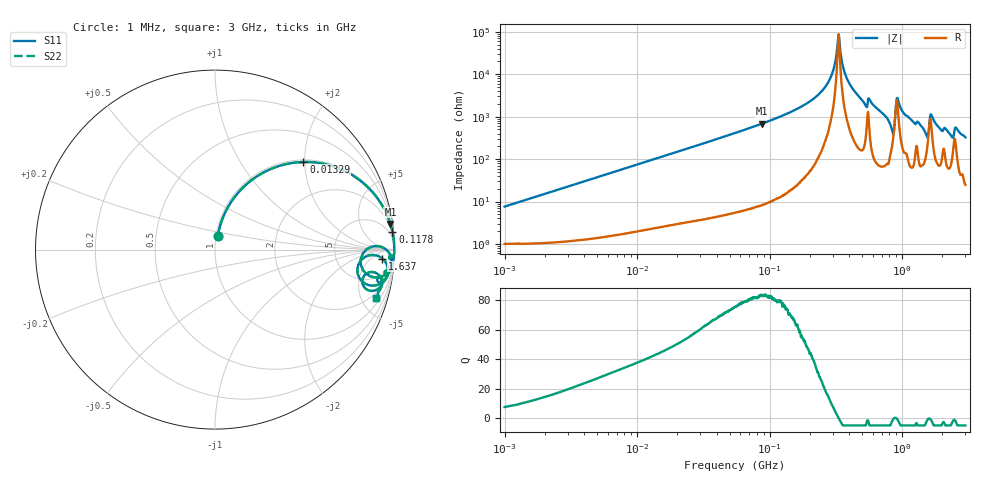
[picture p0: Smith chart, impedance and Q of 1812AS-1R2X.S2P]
!s-Parameter Generated by FASTRON Sdn. Bhd.
!FASTRON P/N : 1812AS-1R2X
!Keysight Technologies,E4991B,MY54100416,A.01.15
!Date created: Fri Oct 13 15:28:02 2023
!Version  : Rev00 Fri Oct 13 15:28:02 2023
!Data & Calibration Information:
!Freq	S11	S21	S12	S22
!PortZ  Port1:50+j0  Port2:50+j0
!When reading, reference impedance value at option line is always used.
! Remarks : This data is being provided solely for informational purposes.
# Hz S dB R 50
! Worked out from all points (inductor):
!   1601 points, 1 MHz to 3 GHz, reference 50 ohm
!   read as one part in series: L = 1.2 uH near 1.041 MHz
!   highest Q = 83.2 at 87.23 MHz (marker M1), where L = 1.25 uH
!   self-resonance near 330.2 MHz
!   S11 on the Smith chart (normalised r, x): 1 MHz: 1.02, +0.15; 13.29 MHz: 1.05, +1.97; 117.8 MHz: 1, +20; 1.637 GHz: 18, -14; 3 GHz: 1.50, -6.53
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1000000  -22.48 78.1  -0.11 -4.3  -0.11 -4.3  -22.48 78.1
3804036  -11.33 71.8  -0.44 -15.7  -0.44 -15.7  -11.33 71.8
1.329061e7  -3.18 44.7  -3.05 -43.9  -3.05 -43.9  -3.18 44.7
1.447069e7  -2.82 42.4  -3.42 -46.3  -3.42 -46.3  -2.82 42.4
5.477226e7  -0.28 13.6  -12.57 -75.6  -12.57 -75.6  -0.28 13.6
8.723049e7  -0.11 8.3  -16.79 -81.0  -16.79 -81.0  -0.11 8.3
1.17777e8  -0.06 5.8  -19.88 -83.5  -19.88 -83.5  -0.06 5.8
2.083556e8  -0.02 2.3  -27.90 -86.3  -27.90 -86.3  -0.02 2.3
2.827291e8  -0.01 0.8  -37.32 -84.7  -37.32 -84.7  -0.01 0.8
3.318279e8  -0.01 -0.0  -58.76 2.8  -58.76 2.8  -0.01 -0.0
3.685956e8  -0.01 -0.5  -40.70 81.5  -40.70 81.5  -0.01 -0.5
4.177151e8  -0.01 -1.2  -33.71 84.6  -33.71 84.6  -0.01 -1.2
5.232078e8  -0.06 -2.9  -26.00 80.5  -26.00 80.5  -0.06 -2.9
5.753936e8  -0.05 -2.4  -27.35 80.9  -27.35 80.9  -0.05 -2.4
7.925923e8  -0.18 -7.1  -18.13 76.7  -18.13 76.7  -0.18 -7.1
8.501091e8  -1.38 -9.1  -13.66 40.5  -13.66 40.5  -1.38 -9.1
9.302341e8  -0.19 -1.9  -28.13 55.5  -28.13 55.5  -0.19 -1.9
1.511446e9  -0.86 -12.8  -12.69 59.8  -12.69 59.8  -0.86 -12.8
1.637435e9  -0.59 -3.1  -21.55 36.5  -21.55 36.5  -0.59 -3.1
2.335937e9  -0.76 -14.5  -11.87 63.7  -11.87 63.7  -0.76 -14.5
2.568929e9  -0.57 -9.7  -15.12 64.2  -15.12 64.2  -0.57 -9.7
3e9  -0.57 -16.6  -10.88 69.1  -10.88 69.1  -0.57 -16.6
